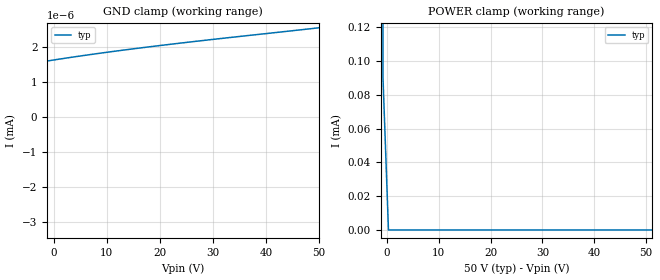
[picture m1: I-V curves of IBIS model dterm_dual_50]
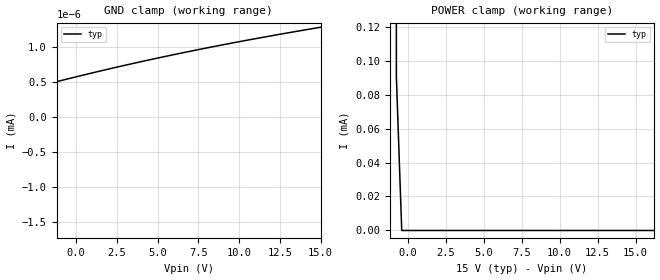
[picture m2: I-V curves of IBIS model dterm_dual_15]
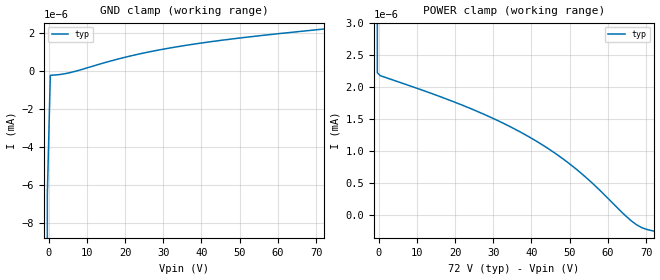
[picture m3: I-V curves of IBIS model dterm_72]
|Texas Instruments Incorporated
|tmux8211, 100V 4 channel 1:1 switch
[IBIS Ver]   4.1
[File name]   tmux8211.ibs
[Date]   07/06/21
[File Rev]   1.0
[Source]
| Texas Instruments Incorporated.
| ASC-INT-MPD
| 12500 TI Blvd
| Dallas, TX - 75243
[Notes]   Revision History:
| Rev 1.0: 07/06/21
| - Initial version of the model
| - Model generated from simulations in SPECTRE
| - C_comp although listed in numerical order of value are
|   obtained from varying PVT conditions. For PVT conditions for
|   each specific value refer the buffer description under
|   respective [Model]. IBIS model user is responsible for using
|   appropriate C_comp to simulate for Signal Integrity.
[Disclaimer]
| This model is designed as an aid for customers of Texas Instruments.
| TI and its licensors and suppliers make no warranties, either expressed
| or implied, with respect to this  model, including the warranties of
| merchantability or fitness for a particular purpose. The model is
| provided solely on an "as is" basis. The entire risk as to its quality
| and performance is with the customer.
| This model is subject to change without notice. Texas Instruments
| Incorporated is not responsible for updating this model.
[Copyright]
(C) Copyright 2021 Texas Instruments Incorporated.All rights reserved.
|  Component TMUX8211PW 16-pin - PW package
|  Part # TMUX8211PW
[Component]   TMUX8211PW
[Manufacturer]  TI
[Package]
|   typ   min   max
R_pkg   0.14389   NA   NA
L_pkg   1.96144nH   NA   NA
C_pkg   0.37623pF   NA   NA
[Pin]   signal_name   model_name
   1   S1   sterm
   2   D1   dterm
   3   SEL1   inbuf
   4   VSS   POWER
   5   GND   GND
   6   SEL4   inbuf
   7   D4   dterm
   8   S4   sterm
   9   S3   sterm
   10   D3   dterm
   11   SEL3   inbuf
   12   NC   NC
   13   VDD   POWER
   14   SEL2   inbuf
   15   D2   dterm
   16   S2   sterm
[Series Switch Groups]
On 1 /
On 2 /
On 3 /
On 4 /
Off 1 2 3 4 /
[Series Pin Mapping]  pin_2 model_name function_table_group
|   1   2   switch_dual_50   1
|   8   7   switch_dual_50   2
|   9  10   switch_dual_50   3
|  16  15   switch_dual_50   4
|   1   2   switch_dual_15   1
|   8   7   switch_dual_15   2
|   9  10   switch_dual_15   3
|  16  15   switch_dual_15   4
|   1   2   switch_72   1
|   8   7   switch_72   2
|   9  10   switch_72   3
|  16  15   switch_72   4
|   1   2   switch_100   1
|   8   7   switch_100   2
|   9  10   switch_100   3
|  16  15   switch_100   4
  1   2   switch_dual_36   1
  8   7   switch_dual_36   2
  9  10   switch_dual_36   3
  16  15   switch_dual_36   4
|  Component TMUX8211RUM 16-pin - RUM package
|  Part # TMUX8211RUM
[Component]   TMUX8211RUM
[Manufacturer]  TI
[Package]
|   typ   min   max
R_pkg   0.1   NA   NA
L_pkg   1.0nH   NA   NA
C_pkg   0.2pF   NA   NA
[Pin]   signal_name   model_name
   1   VSS   POWER
   2   SEL1   inbuf
   3   GND   GND
   4   SEL4   inbuf
   5   D4   dterm
   6   S4   sterm
   7   S3   sterm
   8   D3   dterm
   9   VDD   POWER
   10   NC   NC
   11   SEL3   inbuf
   12   SEL2   inbuf
   13   D2   dterm
   14   S2   sterm
   15   S1   sterm
   16   D1   dterm
[Series Switch Groups]
On 1 /
On 2 /
On 3 /
On 4 /
Off 1 2 3 4 /
[Series Pin Mapping]  pin_2 model_name function_table_group
|  15  16   switch_dual_50   1
|  14  13   switch_dual_50   2
|   7   8   switch_dual_50   3
|   6   5   switch_dual_50   4
|  15  16   switch_dual_15   1
|  14  13   switch_dual_15   2
|   7   8   switch_dual_15   3
|   6   5   switch_dual_15   4
|  15  16   switch_72   1
|  14  13   switch_72   2
|   7   8   switch_72   3
|   6   5   switch_72   4
|  15  16   switch_100   1
|  14  13   switch_100   2
|   7   8   switch_100   3
|   6   5   switch_100   4
  15  16   switch_dual_36   1
  14  13   switch_dual_36   2
   7   8   switch_dual_36   3
   6   5   switch_dual_36   4
[Model Selector] dterm
dterm_dual_50 Use for operation at +/-50V
dterm_dual_15 Use for operation at +/-15V
dterm_72 Use for operation at 72V
dterm_100 Use for operation at 100V
dterm_dual_36 Use for operation at +/-36V
[Model Selector] sterm
sterm_dual_50 Use for operation at +/-50V
sterm_dual_15 Use for operation at +/-15V
sterm_72 Use for operation at 72V
sterm_100 Use for operation at 100V
sterm_dual_36 Use for operation at +/-36V
[Model Selector] inbuf
inbuf_dual_50 Use for operation at +/-50V
inbuf_dual_15 Use for operation at +/-15V
inbuf_72 Use for operation at 72V
inbuf_100 Use for operation at 100V
inbuf_dual_36 Use for operation at +/-36V
| switch_dual_50
[Model]   switch_dual_50
Model_type   Series_switch
|   typ   min   max
C_comp   1.008417e-11   NA   NA
[Voltage Range]   50   NA   NA
[Power Clamp Reference]   50   NA   NA
[Temperature Range]   27   NA   NA
[On]
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[Off]
|   typ   min   max
[R Series]   10G   NA   NA
| switch_dual_15
[Model]   switch_dual_15
Model_type   Series_switch
|   typ   min   max
C_comp   1.008417e-11   NA   NA
[Voltage Range]   15   NA   NA
[Power Clamp Reference]   15   NA   NA
[Temperature Range]   27   NA   NA
[On]
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[Off]
|   typ   min   max
[R Series]   10G   NA   NA
| switch_72
[Model]   switch_72
Model_type   Series_switch
|   typ   min   max
C_comp   1.008417e-11   NA   NA
[Voltage Range]   72   NA   NA
[Power Clamp Reference]   72   NA   NA
[Temperature Range]   27   NA   NA
[On]
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[Off]
|   typ   min   max
[R Series]   10G   NA   NA
| switch_100
[Model]   switch_100
Model_type   Series_switch
|   typ   min   max
C_comp   1.008417e-11   NA   NA
[Voltage Range]   100   NA   NA
[Power Clamp Reference]   100   NA   NA
[Temperature Range]   27   NA   NA
[On]
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[Off]
|   typ   min   max
[R Series]   10G   NA   NA
| switch_dual_36
[Model]   switch_dual_36
Model_type   Series_switch
|   typ   min   max
C_comp   1.008417e-11   NA   NA
[Voltage Range]   36   NA   NA
[Power Clamp Reference]   36   NA   NA
[Temperature Range]   27   NA   NA
[On]
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[Off]
|   typ   min   max
[R Series]   10G   NA   NA
| Models and submodels in the file (20): dterm_dual_50 (Terminator), dterm_dual_15 (Terminator), dterm_72 (Terminator), dterm_100 (Terminator), dterm_dual_36 (Terminator), switch_dual_50 (Series_switch), switch_dual_15 (Series_switch), switch_72 (Series_switch), switch_100 (Series_switch), switch_dual_36 (Series_switch), sterm_dual_50 (Terminator), sterm_dual_15 (Terminator), sterm_72 (Terminator), sterm_100 (Terminator), sterm_dual_36 (Terminator), inbuf_dual_50 (Input), inbuf_dual_15 (Input), inbuf_72 (Input), inbuf_100 (Input), inbuf_dual_36 (Input)
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| dterm_dual_50
[Model]   dterm_dual_50
Model_type   Terminator
|   typ   min   max
C_comp   6.362683e-12   NA   NA
[Voltage Range]   50   NA   NA
[Temperature Range]   27   NA   NA
[Power Clamp Reference]   50   NA   NA
[GND Clamp Reference]   0   NA   NA
[GND Clamp]
|   Voltage   I(typ)   I(min)   I(max)
-55V      -1.446A    NA         NA
-50.76V   -603uA     NA         NA
-49.7V    -323.1pA   NA         NA
-46.52V   -262.9pA   NA         NA
-44.39V   -180.1pA   NA         NA
-32.73V   484.9pA    NA         NA
-25.3V    839.6pA    NA         NA
-17.88V   1.124nA    NA         NA
-10.45V   1.359nA    NA         NA
151.5mV   1.635nA    NA         NA
12.88V    1.909nA    NA         NA
50V       2.552nA    NA         NA
[POWER Clamp]
|   Voltage   I(typ)   I(min)   I(max)
-5V       744mA      NA         NA
-1.818V   145.4mA    NA         NA
-757.6mV  90.5uA     NA         NA
303mV     2.547nA    NA         NA
100V      -327pA     NA         NA
| dterm_dual_15
[Model]   dterm_dual_15
Model_type   Terminator
|   typ   min   max
C_comp   6.362683e-12   NA   NA
[Voltage Range]   15   NA   NA
[Temperature Range]   27   NA   NA
[Power Clamp Reference]   15   NA   NA
[GND Clamp Reference]   0   NA   NA
[GND Clamp]
|   Voltage   I(typ)   I(min)   I(max)
-20V      -1.446A    NA         NA
-15.4V    -92.79nA   NA         NA
-15.05V   -116.5pA   NA         NA
-11.87V   -61.1pA    NA         NA
-9.394V   32.33pA    NA         NA
-6.919V   164pA      NA         NA
151.5mV   584.6pA    NA         NA
4.04V     795.7pA    NA         NA
9.343V    1.05nA     NA         NA
15V       1.286nA    NA         NA
[POWER Clamp]
|   Voltage   I(typ)   I(min)   I(max)
-5V       744mA      NA         NA
-1.111V   26.13mA    NA         NA
-757.6mV  90.5uA     NA         NA
-404mV    1.662nA    NA         NA
30V       -115.6pA   NA         NA
| dterm_72
[Model]   dterm_72
Model_type   Terminator
|   typ   min   max
C_comp   6.362683e-12   NA   NA
[Voltage Range]   72   NA   NA
[Temperature Range]   27   NA   NA
[Power Clamp Reference]   72   NA   NA
[GND Clamp Reference]   0   NA   NA
[GND Clamp]
|   Voltage   I(typ)   I(min)   I(max)
-5V       -1.446A    NA         NA
-1.111V   -28.81mA   NA         NA
-333.3mV  -6.504nA   NA         NA
444.4mV   -237.3pA   NA         NA
5.111V    -118.5pA   NA         NA
20.67V    741.2pA    NA         NA
33.11V    1.243nA    NA         NA
48.67V    1.686nA    NA         NA
72V       2.19nA     NA         NA
[POWER Clamp]
|   Voltage   I(typ)   I(min)   I(max)
-5V       744mA      NA         NA
-1.111V   26.13mA    NA         NA
-333.3mV  2.226nA    NA         NA
444.4mV   2.181nA    NA         NA
23.78V    1.675nA    NA         NA
32.33V    1.447nA    NA         NA
39.33V    1.227nA    NA         NA
45.56V    996.4pA    NA         NA
51.78V    719.6pA    NA         NA
66.56V    -103.6pA   NA         NA
68.89V    -189.6pA   NA         NA
72V       -243pA     NA         NA
